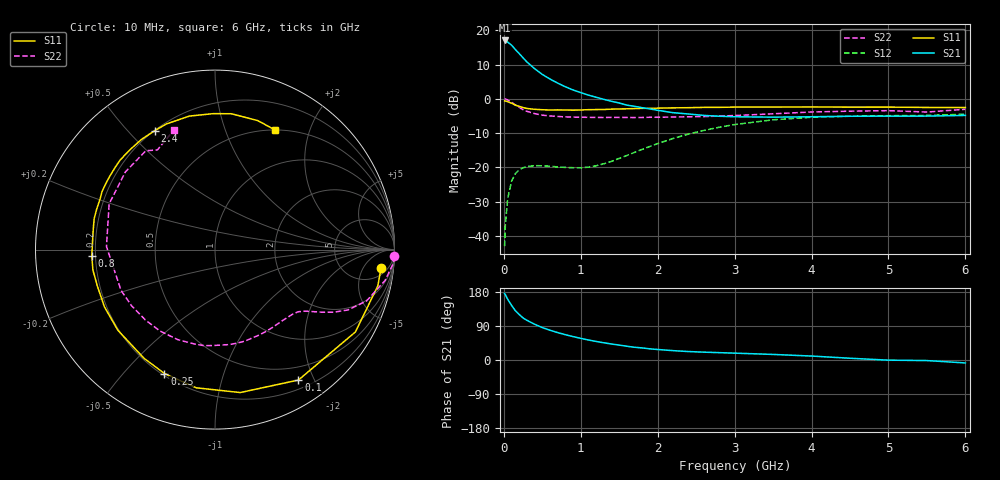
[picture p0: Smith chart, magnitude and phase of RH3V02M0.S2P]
! SIEMENS Small Signal Semiconductors
! BFR106
! Si NPN RF Bipolar Junction Transistor in SOT23
! VCE = 3 V  IC = 2 mA
! Common Emitter S-Parameters:  August  1996
# GHz  S  MA  R  50
!  f  S11  S21  S12  S22
! GHz  MAG  ANG  MAG  ANG  MAG  ANG  MAG  ANG
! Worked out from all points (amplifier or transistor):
!   36 points, 10 MHz to 6 GHz, reference 50 ohm
!   highest |S21| = 17.0 dB at 10 MHz (marker M1)
!   |S21| within 3 dB of that: start of sweep to 164.8 MHz
!   unconditionally stable (mu >= 1): 779.1 MHz to 2.027 GHz; 3.531 GHz to end of sweep
!   at 250 MHz: K = 0.32, MSG = 16.0 dB, |S12| = -20.1 dB
!   at 1.4 GHz: K = 1.28, MAG = 5.6 dB, |S12| = -18.2 dB
!   at 6 GHz: K = 1.02, MAG = -1.1 dB, |S12| = -4.5 dB
!   S11 on the Smith chart (normalised r, x): 10 MHz: 8, -13; 100 MHz: 0.31, -1.78; 250 MHz: 0.21, -0.65; 800 MHz: 0.19, -0.03; 2.4 GHz: 0.20, +0.60; 6 GHz: 0.50, +1.50
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0.01  0.9313 -6.2  7.099 175.4  0.0071 88.0  0.9985 -2.2
0.02  0.9293 -12.6  7.027 172.2  0.0147 81.2  0.9965 -4.4
0.05  0.9069 -30.4  6.713 160.2  0.0351 72.9  0.963 -10.3
0.1  0.8627 -57.4  6.072 144.3  0.0627 59.5  0.8918 -18.7
0.15  0.8087 -80.0  5.232 129.9  0.0811 48.3  0.8138 -24.4
0.2  0.7771 -97.7  4.566 120.0  0.0922 41.1  0.7495 -27.7
0.25  0.7457 -112.2  3.959 111.0  0.0989 35.2  0.6939 -30.2
0.3  0.7231 -123.2  3.446 104.7  0.1028 31.7  0.6574 -31.8
0.4  0.7034 -140.3  2.752 94.3  0.106 26.6  0.6082 -34.3
0.5  0.6937 -152.6  2.267 85.6  0.1056 24.4  0.5781 -36.8
0.6  0.6863 -162.8  1.943 78.5  0.1041 24.2  0.5624 -39.8
0.8  0.6873 -177.0  1.499 66.8  0.1 27.9  0.5453 -46.6
1.1  0.695 165.6  1.133 52.8  0.1008 42.0  0.5371 -58.4
1.6  0.7152 144.6  0.809 36.2  0.1493 63.6  0.5352 -81.3
2.2  0.7382 123.6  0.628 24.7  0.2638 64.2  0.5429 -112.4
2.4  0.7428 116.9  0.601 22.3  0.3059 61.0  0.5474 -124.0
3  0.7575 100.9  0.548 18.1  0.4217 48.0  0.5706 -156.6
3.5  0.7576 90.7  0.54 14.7  0.4944 36.1  0.6049 178.4
4.5  0.7559 76.8  0.557 4.6  0.558 14.9  0.6606 139.1
5  0.7571 71.7  0.559 -0.4  0.5675 7.0  0.6722 125.0
5.5  0.7487 66.8  0.56 -1.5  0.5727 3.3  0.6415 120.0
6  0.7457 63.3  0.573 -7.8  0.5958 -4.5  0.704 109.0
